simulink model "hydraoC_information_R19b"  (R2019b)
settings: Solver=VariableStepAuto  StartTime=0.0  StopTime=inf  FixedStep=1e-3  RelTol=1e-3
libraries: fl_lib x33, ee_lib x10, nesl_utility x6, simulink x2, sh_lib x1

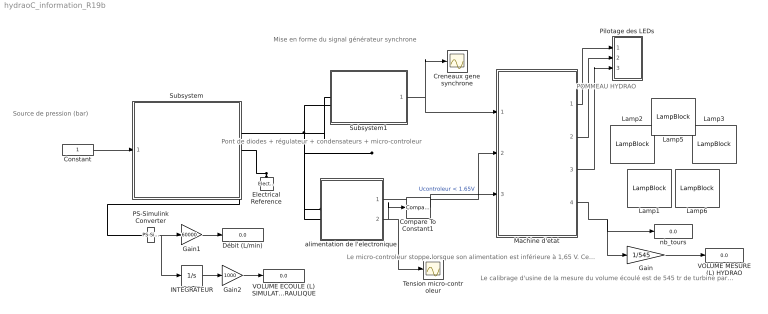
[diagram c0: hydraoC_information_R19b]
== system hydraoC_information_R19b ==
  note: POMMEAU HYDRAO
  note: Le calibrage d'usine de la mesure du volume écoulé est de 545 tr de turbine par litre.
  note: Mise en forme du signal générateur synchrone
  note: Pont de diodes + régulateur + condensateurs + micro-controleur
  note: Source de pression (bar)
  note: Le micro-controleur stoppe lorsque son alimentation est inférieure à 1,65 V. Cela entraine une perte des informations et un redémarrage en situation initiale au prochain écoulement
  Compare To Constant1 : simulink/Logic and Bit Operations/Compare To Constant  relop=<  const=1.65  OutDataTypeStr=boolean
  Constant : Constant
  Creneaux gene synchrone : Scope
  Débit (L/min) : Display
  Electrical Reference : fl_lib/Electrical/Electrical Elements/Electrical Reference
  Gain : Gain  Gain=1/545
  Gain1 : Gain  Gain=60000
  Gain2 : Gain  Gain=1000
  INTEGRATEUR : Integrator
  Lamp{1..3,5..6} (5 alike) : LampBlock
  Machine d'etat : Stateflow chart  TreatAsAtomicUnit=on
  PS-Simulink Converter : nesl_utility/PS-Simulink Converter  PhysicalDomain=network_engine_domain  SubClassName=ps_output  LeftPortType=input  RightPortType=output  PseudoPeriodic=off  Frequencies=[]  Unit=inherit  AffineConversion=off
  Pilotage des LEDs : Subsystem
  Subsystem : Subsystem
  Subsystem1 : Subsystem
  Tension micro-controleur : Scope
  VOLUME ECOULE (L) SIMULATION HYDRAULIQUE : Display
  VOLUME MESURE (L) HYDRAO : Display
  alimentation de l'electronique : Subsystem
  nb_tours : Display
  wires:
  Machine d'etat/2(LED_V) -> Pilotage des LEDs/2(V)
  Machine d'etat/3(LED_B) -> Pilotage des LEDs/3(B)
  Machine d'etat/1(LED_R) -> Pilotage des LEDs/1(R)
  Machine d'etat/4(nb_tours) -> nb_tours/1, Gain/1
  alimentation de l'electronique/2(Ucontroleur) -> Tension micro-controleur/1, Compare To Constant1/1
  Constant/1 -> Subsystem/1(In1)
  Subsystem1/1(Creneaux_gene_alt) -> Machine d'etat/1(creneau_gene), Creneaux gene synchrone/1
  alimentation de l'electronique/1(Image_Upuiss) -> Machine d'etat/2(image_Upuiss)
  Compare To Constant1/1 -> Machine d'etat/3(alim_LOW)  "Ucontroleur < 1.65V"
  Gain/1 -> VOLUME MESURE (L) HYDRAO/1
  PS-Simulink Converter/1 -> INTEGRATEUR/1, Gain1/1
  Gain1/1 -> Débit (L/min)/1
  Gain2/1 -> VOLUME ECOULE (L) SIMULATION HYDRAULIQUE/1
  INTEGRATEUR/1 -> Gain2/1
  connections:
  Subsystem/RConn1 -- alimentation de l'electronique/LConn1 -- Subsystem1/LConn1
  Electrical Reference/LConn1 -- Subsystem/RConn2 -- Subsystem1/LConn2 -- alimentation de l'electronique/LConn2
  Subsystem/RConn3 -- PS-Simulink Converter/LConn1

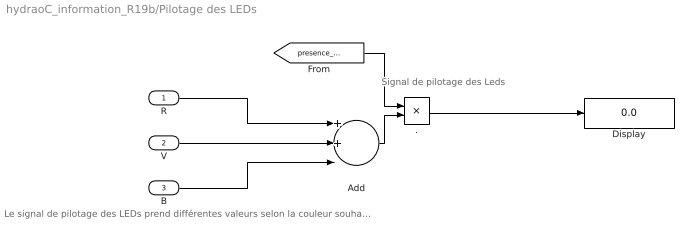
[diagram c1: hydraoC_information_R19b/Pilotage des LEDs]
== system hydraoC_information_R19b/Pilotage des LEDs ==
  note: Signal de pilotage des Leds
  note: Le signal de pilotage des LEDs prend différentes valeurs selon la couleur souhaitée Vmot est un booleen qui vaut 0L si la tension aux bornes du pont de diodes les LEDs ne peuvent s'éclairer que si le pont est alimenté donc si la turbine tourne
  R : Inport
  V : Inport  Port=2
  B : Inport  Port=3
  . : Product
  Add : Sum  Inputs=3
  Display : Display
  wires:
  B/1 -> Add/3
  ./1 -> Display/1
  R/1 -> Add/1
  V/1 -> Add/2
  Add/1 -> ./2
  [presence_Upuiss] -> ./1

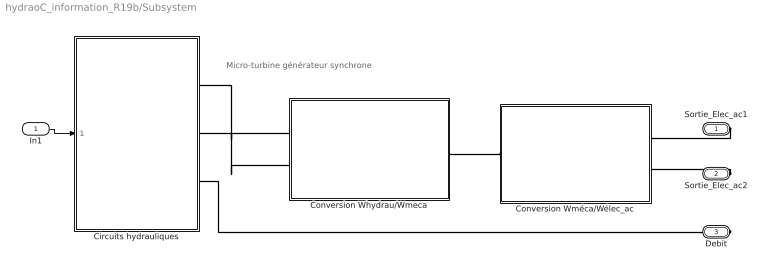
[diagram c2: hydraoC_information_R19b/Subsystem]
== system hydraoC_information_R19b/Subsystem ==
  note: Micro-turbine générateur synchrone
  In1 : Inport
  Circuits hydrauliques : Subsystem
  Conversion Whydrau/Wmeca : Subsystem
  Conversion Wméca/Wélec_ac : Subsystem
  Sortie_Elec_ac1 : PMIOPort  Side=Right
  Sortie_Elec_ac2 : PMIOPort  Port=2  Side=Right
  Debit : PMIOPort  Port=3  Side=Right
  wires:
  In1/1 -> Circuits hydrauliques/1(Pression source)
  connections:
  Sortie_Elec_ac1/RConn1 -- Conversion Wméca/Wélec_ac/RConn1
  Circuits hydrauliques/RConn2 -- Conversion Whydrau/Wmeca/LConn2
  Conversion Whydrau/Wmeca/RConn1 -- Conversion Wméca/Wélec_ac/LConn1
  Circuits hydrauliques/RConn1 -- Conversion Whydrau/Wmeca/LConn1
  Sortie_Elec_ac2/RConn1 -- Conversion Wméca/Wélec_ac/RConn2
  Circuits hydrauliques/RConn3 -- Debit/RConn1

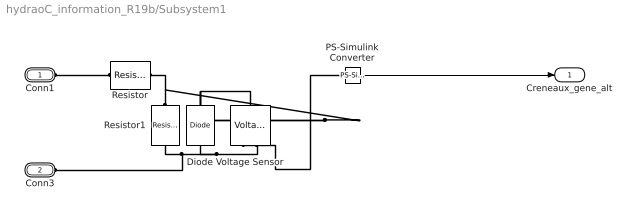
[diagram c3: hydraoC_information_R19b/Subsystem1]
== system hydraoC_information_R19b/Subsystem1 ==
  Diode : ee_lib/Semiconductors & Converters/Diode  ModelType=ee.enum.diode.modelType.pwl  Vf=0.6 V  Ron=0.3 Ohm  Goff=1e-8 S  prmExp=ee.enum.diode.expParam.useTwo  I12=[.0137, .545] A  V12=[.6, .7] V  IS=1e-12 A  ec=1  I1=0.0137 A  V1=0.6 V  RS=0 Ohm  Tmeas=25 degC  N_series=1  N_parallel=1  Rz=0.3 Ohm  BV=3 V  C_param=ee.enum.diode.capParam.fixed  CJ=5 pF  CJ0=5 pF  VJ=1 V  Mgrad=0.5  Vvec=[.1, 10, 100] V  Cvec=[3.5, 1, .4] pF  FC=0.5  Q_param=ee.enum.diode.recoveryParam.off  iRM=-7.15 A  iF=4 A  didt=-750 A/us  trr_factor=3  trr=115 ns  Qrr=1500 s*uA  TT=50 ns  tau=100 ns  T_param=ee.enum.diode.temperatureParam.off  IS_T2=1.25e-7 A  I1_T2=0.245 A  V1_T2=0.5 V  Tmeas2=125 degC  EG_param=ee.enum.diode.egapParam.material_si  EG=1.11 eV  XTI_param=ee.enum.diode.xtiParam.pn  XTI=3  dBVdT=0 V/K  Tdevice=25 degC  i_specify=off  i_priority=None  i=0 A  i_nominal_specify=off  i_nominal_unit=A  i_nominal_value=1  v_specify=off  v_priority=None  v=0 V  v_nominal_specify=off  v_nominal_unit=V  v_nominal_value=1  i_capacitor_specify=off  i_capacitor_priority=None  i_capacitor=0 A  i_capacitor_nominal_specify=off  i_capacitor_nominal_unit=A  i_capacitor_nominal_value=1  v_capacitor_specify=off  v_capacitor_priority=None  v_capacitor=0 V  v_capacitor_nominal_specify=off  v_capacitor_nominal_unit=V  v_capacitor_nominal_value=1  power_dissipated_specify=off  power_dissipated_priority=None  power_dissipated=0 W  power_dissipated_nominal_specify=off  power_dissipated_nominal_unit=W  power_dissipated_nominal_value=1  thermal_network_parameterization=ee.enum.thermalNetworkTopology.cauer  Rth=[0, 10] K/W  Rth_Foster=[4, 6] K/W  thermal_mass_parameterization=ee.enum.thermalNetwork.timeconstant  thermal_mass=[0, 1] J/K  thermal_mass_Foster=[1.5, 3] J/K  thermal_time_constant=[0, 10] s  thermal_time_constant_Foster=[6, 18] s  thermal_mass_initial_temperatures=[25, 25] degC
  PS-Simulink Converter : nesl_utility/PS-Simulink Converter  PhysicalDomain=network_engine_domain  SubClassName=ps_output  LeftPortType=input  RightPortType=output  PseudoPeriodic=off  Frequencies=[]  Unit=inherit  AffineConversion=off
  Resistor : fl_lib/Electrical/Electrical Elements/Resistor  R=10 kOhm  i_specify=off  i_priority=None  i=0 A  i_nominal_specify=off  i_nominal_unit=A  i_nominal_value=1  v_specify=off  v_priority=None  v=0 V  v_nominal_specify=off  v_nominal_unit=V  v_nominal_value=1
  Resistor1 : fl_lib/Electrical/Electrical Elements/Resistor  R=330 kOhm  i_specify=off  i_priority=None  i=0 A  i_nominal_specify=off  i_nominal_unit=A  i_nominal_value=1  v_specify=off  v_priority=None  v=0 V  v_nominal_specify=off  v_nominal_unit=V  v_nominal_value=1
  Voltage Sensor : fl_lib/Electrical/Electrical Sensors/Voltage Sensor
  Conn1 : PMIOPort  Side=Left
  Conn3 : PMIOPort  Port=2  Side=Left
  Creneaux_gene_alt : Outport
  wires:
  PS-Simulink Converter/1 -> Creneaux_gene_alt/1
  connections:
  Resistor1/LConn1 -- Resistor/RConn1 -- Voltage Sensor/LConn1 -- Diode/RConn1
  Voltage Sensor/RConn2 -- Diode/LConn1 -- Conn3/RConn1 -- Resistor1/RConn1
  Resistor/LConn1 -- Conn1/RConn1
  PS-Simulink Converter/LConn1 -- Voltage Sensor/RConn1

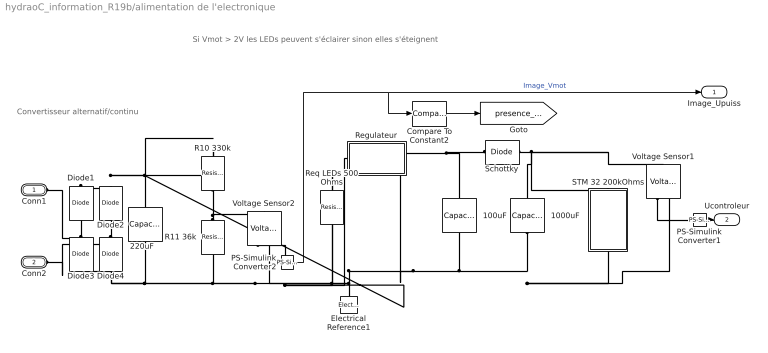
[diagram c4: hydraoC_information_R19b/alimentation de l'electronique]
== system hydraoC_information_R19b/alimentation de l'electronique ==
  note: Convertisseur alternatif/continu
  note: Si Vmot > 2V les LEDs peuvent s'éclairer sinon elles s'éteignent
  " 1000uF" : ee_lib/Passive/Capacitor  cap_option=0  c=1000 uF  Cvec=[1e-05, 1e-06] F  Vvec=[0, 10] V  CV_table_symmetry=1  f_vec=[1, 10] kHz  DFext_vec=[.8, 1.2]  C_tol=5  enable_C_tol=0  tol_distribution=1  nSigma=4  r=1e-6 Ohm  g=0 1/Ohm  averaging_period=0 s  enable_operating_limits=0  operating_limit_action=2  max_working_voltage_range=[-25, 25] V  power_rating=1 W  enable_faults=0  fault_action=1  Cscale_faulted=100  R_faulted=1e-3 Ohm  G_faulted=0 1/Ohm  tau_fault=1e-3 s  enable_temporal_fault=0  t_fault=1 s  enable_behavioral_fault=0  max_permissible_voltage_range=[-100, 100] V  t_fail_on_voltage=1 s  i_specify=off  i_priority=None  i=0 A  i_nominal_specify=off  i_nominal_unit=A  i_nominal_value=1  v_specify=off  v_priority=None  v=0 V  v_nominal_specify=off  v_nominal_unit=V  v_nominal_value=1  vc_specify=off  vc_priority=High  vc=0 V  vc_nominal_specify=off  vc_nominal_unit=V  vc_nominal_value=1
  " 100uF" : ee_lib/Passive/Capacitor  cap_option=0  c=100 uF  Cvec=[1e-05, 1e-06] F  Vvec=[0, 10] V  CV_table_symmetry=1  f_vec=[1, 10] kHz  DFext_vec=[.8, 1.2]  C_tol=5  enable_C_tol=0  tol_distribution=1  nSigma=4  r=1e-6 Ohm  g=0 1/Ohm  averaging_period=0 s  enable_operating_limits=0  operating_limit_action=2  max_working_voltage_range=[-25, 25] V  power_rating=1 W  enable_faults=0  fault_action=1  Cscale_faulted=100  R_faulted=1e-3 Ohm  G_faulted=0 1/Ohm  tau_fault=1e-3 s  enable_temporal_fault=0  t_fault=1 s  enable_behavioral_fault=0  max_permissible_voltage_range=[-100, 100] V  t_fail_on_voltage=1 s  i_specify=off  i_priority=None  i=0 A  i_nominal_specify=off  i_nominal_unit=A  i_nominal_value=1  v_specify=off  v_priority=None  v=0 V  v_nominal_specify=off  v_nominal_unit=V  v_nominal_value=1  vc_specify=off  vc_priority=High  vc=0 V  vc_nominal_specify=off  vc_nominal_unit=V  vc_nominal_value=1
  " 220uF" : ee_lib/Passive/Capacitor  cap_option=0  c=220 uF  Cvec=[1e-05, 1e-06] F  Vvec=[0, 10] V  CV_table_symmetry=1  f_vec=[1, 10] kHz  DFext_vec=[.8, 1.2]  C_tol=5  enable_C_tol=0  tol_distribution=1  nSigma=4  r=1e-6 Ohm  g=0 1/Ohm  averaging_period=0 s  enable_operating_limits=0  operating_limit_action=2  max_working_voltage_range=[-25, 25] V  power_rating=1 W  enable_faults=0  fault_action=1  Cscale_faulted=100  R_faulted=1e-3 Ohm  G_faulted=0 1/Ohm  tau_fault=1e-3 s  enable_temporal_fault=0  t_fault=1 s  enable_behavioral_fault=0  max_permissible_voltage_range=[-100, 100] V  t_fail_on_voltage=1 s  i_specify=off  i_priority=None  i=0 A  i_nominal_specify=off  i_nominal_unit=A  i_nominal_value=1  v_specify=off  v_priority=None  v=0 V  v_nominal_specify=off  v_nominal_unit=V  v_nominal_value=1  vc_specify=off  vc_priority=High  vc=0 V  vc_nominal_specify=off  vc_nominal_unit=V  vc_nominal_value=1
  Compare To Constant2 : simulink/Logic and Bit Operations/Compare To Constant  relop=>  const=0.2  OutDataTypeStr=boolean
  Diode{1..4} (4 alike) : fl_lib/Electrical/Electrical Elements/Diode  Vf=0.3 V  Ron=1 Ohm  Goff=1e-8 1/Ohm  i_specify=off  i_priority=None  i=0 A  i_nominal_specify=off  i_nominal_unit=A  i_nominal_value=1  v_specify=off  v_priority=None  v=0 V  v_nominal_specify=off  v_nominal_unit=V  v_nominal_value=1
  Electrical Reference1 : fl_lib/Electrical/Electrical Elements/Electrical Reference
  PS-Simulink Converter1 : nesl_utility/PS-Simulink Converter  PhysicalDomain=network_engine_domain  SubClassName=ps_output  LeftPortType=input  RightPortType=output  PseudoPeriodic=off  Frequencies=[]  Unit=inherit  AffineConversion=off
  PS-Simulink Converter2 : nesl_utility/PS-Simulink Converter  PhysicalDomain=network_engine_domain  SubClassName=ps_output  LeftPortType=input  RightPortType=output  PseudoPeriodic=off  Frequencies=[]  Unit=inherit  AffineConversion=off
  R10 330k : fl_lib/Electrical/Electrical Elements/Resistor  R=330 kOhm  i_specify=off  i_priority=None  i=0 A  i_nominal_specify=off  i_nominal_unit=A  i_nominal_value=1  v_specify=off  v_priority=None  v=0 V  v_nominal_specify=off  v_nominal_unit=V  v_nominal_value=1
  R11 36k : fl_lib/Electrical/Electrical Elements/Resistor  R=36 kOhm  i_specify=off  i_priority=None  i=0 A  i_nominal_specify=off  i_nominal_unit=A  i_nominal_value=1  v_specify=off  v_priority=None  v=0 V  v_nominal_specify=off  v_nominal_unit=V  v_nominal_value=1
  Regulateur : Subsystem
  Req LEDs 500 Ohms : fl_lib/Electrical/Electrical Elements/Resistor  R=500 Ohm  i_specify=off  i_priority=None  i=0 A  i_nominal_specify=off  i_nominal_unit=A  i_nominal_value=1  v_specify=off  v_priority=None  v=0 V  v_nominal_specify=off  v_nominal_unit=V  v_nominal_value=1
  STM 32 200kOhms : Subsystem
  Schottky : ee_lib/Semiconductors & Converters/Diode  ModelType=ee.enum.diode.modelType.pwl  Vf=0.3 V  Ron=0.3 Ohm  Goff=1e-8 S  prmExp=ee.enum.diode.expParam.useTwo  I12=[.0137, .545] A  V12=[.6, .7] V  IS=1e-12 A  ec=1  I1=0.0137 A  V1=0.6 V  RS=0 Ohm  Tmeas=25 degC  N_series=1  N_parallel=1  Rz=0.3 Ohm  BV=100 V  C_param=ee.enum.diode.capParam.fixed  CJ=5 pF  CJ0=5 pF  VJ=1 V  Mgrad=0.5  Vvec=[.1, 10, 100] V  Cvec=[3.5, 1, .4] pF  FC=0.5  Q_param=ee.enum.diode.recoveryParam.off  iRM=-7.15 A  iF=4 A  didt=-750 A/us  trr_factor=3  trr=115 ns  Qrr=1500 s*uA  TT=50 ns  tau=100 ns  T_param=ee.enum.diode.temperatureParam.off  IS_T2=1.25e-7 A  I1_T2=0.245 A  V1_T2=0.5 V  Tmeas2=125 degC  EG_param=ee.enum.diode.egapParam.material_si  EG=1.11 eV  XTI_param=ee.enum.diode.xtiParam.pn  XTI=3  dBVdT=0 V/K  Tdevice=25 degC  i_specify=off  i_priority=None  i=0 A  i_nominal_specify=off  i_nominal_unit=A  i_nominal_value=1  v_specify=off  v_priority=None  v=0 V  v_nominal_specify=off  v_nominal_unit=V  v_nominal_value=1  i_capacitor_specify=off  i_capacitor_priority=None  i_capacitor=0 A  i_capacitor_nominal_specify=off  i_capacitor_nominal_unit=A  i_capacitor_nominal_value=1  v_capacitor_specify=off  v_capacitor_priority=None  v_capacitor=0 V  v_capacitor_nominal_specify=off  v_capacitor_nominal_unit=V  v_capacitor_nominal_value=1  power_dissipated_specify=off  power_dissipated_priority=None  power_dissipated=0 W  power_dissipated_nominal_specify=off  power_dissipated_nominal_unit=W  power_dissipated_nominal_value=1  thermal_network_parameterization=ee.enum.thermalNetworkTopology.cauer  Rth=[0, 10] K/W  Rth_Foster=[4, 6] K/W  thermal_mass_parameterization=ee.enum.thermalNetwork.timeconstant  thermal_mass=[0, 1] J/K  thermal_mass_Foster=[1.5, 3] J/K  thermal_time_constant=[0, 10] s  thermal_time_constant_Foster=[6, 18] s  thermal_mass_initial_temperatures=[25, 25] degC
  Voltage Sensor1 : fl_lib/Electrical/Electrical Sensors/Voltage Sensor
  Voltage Sensor2 : fl_lib/Electrical/Electrical Sensors/Voltage Sensor
  Conn1 : PMIOPort  Side=Left
  Conn2 : PMIOPort  Port=2  Side=Left
  Image_Upuiss : Outport
  Ucontroleur : Outport  Port=2
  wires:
  PS-Simulink Converter1/1 -> Ucontroleur/1
  PS-Simulink Converter2/1 -> Compare To Constant2/1, Image_Upuiss/1  "Image_Vmot"
  Compare To Constant2/1 -> [presence_Upuiss]
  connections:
  " 1000uF"/RConn1 -- " 220uF"/RConn1 -- Diode4/LConn1 -- Diode3/LConn1 -- R11 36k/RConn1 -- Voltage Sensor2/RConn2 -- Req LEDs 500 Ohms/RConn1 -- Electrical Reference1/LConn1 -- Regulateur/RConn2 -- " 100uF"/RConn1 -- Voltage Sensor1/RConn2 -- STM 32 200kOhms/RConn1
  Schottky/RConn1 -- " 1000uF"/LConn1 -- STM 32 200kOhms/LConn1 -- Voltage Sensor1/LConn1
  Diode4/RConn1 -- Diode2/LConn1 -- Conn2/RConn1
  Diode1/RConn1 -- R10 330k/LConn1 -- Req LEDs 500 Ohms/LConn1 -- Regulateur/LConn1 -- " 220uF"/LConn1 -- Diode2/RConn1
  Voltage Sensor1/RConn1 -- PS-Simulink Converter1/LConn1
  Regulateur/RConn1 -- " 100uF"/LConn1 -- Schottky/LConn1
  Diode3/RConn1 -- Diode1/LConn1 -- Conn1/RConn1
  PS-Simulink Converter2/LConn1 -- Voltage Sensor2/RConn1
  R11 36k/LConn1 -- Voltage Sensor2/LConn1 -- R10 330k/RConn1

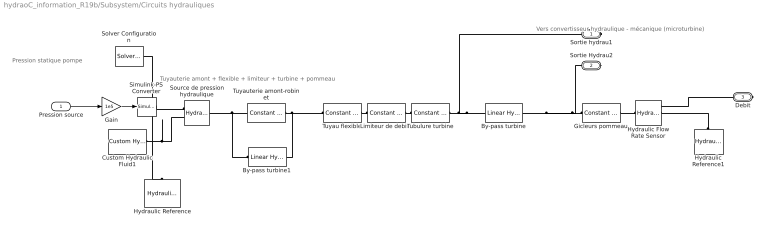
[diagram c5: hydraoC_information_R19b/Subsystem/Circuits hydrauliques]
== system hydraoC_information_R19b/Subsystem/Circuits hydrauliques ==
  note: Pression statique pompe
  note: Tuyauterie amont + flexible + limiteur + turbine + pommeau
  note: Vers convertisseur hydraulique - mécanique (microturbine)
  Pression source : Inport
  By-pass turbine : fl_lib/Hydraulic/Hydraulic Elements/Linear Hydraulic Resistance  Commented=on  resistance=1e0 Pa/(m^3/s)  q_specify=off  q_priority=None  q=0.001 m^3/s  q_nominal_specify=off  q_nominal_unit=m^3/s  q_nominal_value=1  p_specify=off  p_priority=None  p=0 Pa  p_nominal_specify=off  p_nominal_unit=Pa  p_nominal_value=1
  By-pass turbine1 : fl_lib/Hydraulic/Hydraulic Elements/Linear Hydraulic Resistance  Commented=on  resistance=1e0 Pa/(m^3/s)  q_specify=off  q_priority=None  q=0.001 m^3/s  q_nominal_specify=off  q_nominal_unit=m^3/s  q_nominal_value=1  p_specify=off  p_priority=None  p=0 Pa  p_nominal_specify=off  p_nominal_unit=Pa  p_nominal_value=1
  Custom Hydraulic Fluid1 : fl_lib/Hydraulic/Hydraulic Utilities/Custom Hydraulic Fluid  density=994 kg/m^3  viscosity_kin=7.35e-7 m^2/s  bulk=8e8 Pa  alpha=0.005  range_error=2
  Gain : Gain  Gain=1e5
  Gicleurs pommeau : fl_lib/Hydraulic/Hydraulic Elements/Constant Area Hydraulic Orifice  area=20e-6 m^2  C_d=0.4  lam_spec=2  B_lam=0.999  Re_cr=1e0  q_specify=off  q_priority=None  q=0.001 m^3/s  q_nominal_specify=off  q_nominal_unit=m^3/s  q_nominal_value=1  p_specify=off  p_priority=None  p=0 Pa  p_nominal_specify=off  p_nominal_unit=Pa  p_nominal_value=1
  Hydraulic Flow Rate Sensor : fl_lib/Hydraulic/Hydraulic Sensors/Hydraulic Flow Rate Sensor
  Hydraulic Reference : fl_lib/Hydraulic/Hydraulic Elements/Hydraulic Reference
  Hydraulic Reference1 : fl_lib/Hydraulic/Hydraulic Elements/Hydraulic Reference
  Limiteur de debit4 : fl_lib/Hydraulic/Hydraulic Elements/Constant Area Hydraulic Orifice  area=20e-6 m^2  C_d=.5  lam_spec=2  B_lam=0.999  Re_cr=1e0  q_specify=off  q_priority=None  q=0.001 m^3/s  q_nominal_specify=off  q_nominal_unit=m^3/s  q_nominal_value=1  p_specify=off  p_priority=None  p=0 Pa  p_nominal_specify=off  p_nominal_unit=Pa  p_nominal_value=1
  Simulink-PS Converter : nesl_utility/Simulink-PS Converter  PhysicalDomain=network_engine_domain  SubClassName=ps_input  LeftPortType=input  RightPortType=output  PseudoPeriodic=off  Frequencies=[]  NoiseDistribution=none  NoiseParameters=[]  Unit=1  AffineConversion=off  FilteringAndDerivatives=provide  SimscapeFilterOrder=1  InputFilterTimeConstant=0.001  UdotUserProvided=0
  Solver Configuration : nesl_utility/Solver Configuration  PhysicalDomain=network_engine_domain  SubClassName=solver  LeftPortType=input  RightPortType=generic  Tones=[]  Harmonics=[]  SimulateNoise=off  Profile=off  UseLocalSampling=off  EnableSwitchedLinearOptims=on  FrequencyDomain=off  UseCCode=off  RelTol=0.001  AbsTol=1e-06  MinStep=1e-09  ToWorkspace=off  RevertToSquareIcSolve=off  NumHomotopyIterations=100  PhasorMode=off  PhasorModeNumHarmonics=1  DoDC=off  ResidualTolerance=1e-9  UseLocalSolver=off  LocalSolverChoice=NE_BACKWARD_EULER_ADVANCER  LocalSolverSampleTime=0.001  DoFixedCost=off  MaxNonlinIter=3  MaxModeIter=2  LinearAlgebra=Sparse  EquationFormulation=NE_TIME_EF  DelaysMemoryBudget=1024  AutomaticFiltering=on  FilteringTimeConstant=0.001  PartitionStorageMethod=AS_NEEDED  PartitionMemoryBudget=1024  PartitionMethod=FAST
  Source de pression hydraulique : fl_lib/Hydraulic/Hydraulic Sources/Hydraulic Pressure Source
  Tubulure turbine : fl_lib/Hydraulic/Hydraulic Elements/Constant Area Hydraulic Orifice  area=12.7e-6 m^2  C_d=0.81  lam_spec=2  B_lam=0.999  Re_cr=1e0  q_specify=off  q_priority=None  q=0.001 m^3/s  q_nominal_specify=off  q_nominal_unit=m^3/s  q_nominal_value=1  p_specify=off  p_priority=None  p=0 Pa  p_nominal_specify=off  p_nominal_unit=Pa  p_nominal_value=1
  Tuyau flexible : fl_lib/Hydraulic/Hydraulic Elements/Constant Area Hydraulic Orifice  area=41e-6 m^2  C_d=0.25  lam_spec=2  B_lam=2000  Re_cr=1e0  q_specify=off  q_priority=None  q=0.001 m^3/s  q_nominal_specify=off  q_nominal_unit=m^3/s  q_nominal_value=1  p_specify=off  p_priority=None  p=0 Pa  p_nominal_specify=off  p_nominal_unit=Pa  p_nominal_value=1
  Tuyauterie amont-robinet : fl_lib/Hydraulic/Hydraulic Elements/Constant Area Hydraulic Orifice  area=113e-6 m^2  C_d=0.134  lam_spec=2  B_lam=0.999  Re_cr=1e0  q_specify=off  q_priority=None  q=0.001 m^3/s  q_nominal_specify=off  q_nominal_unit=m^3/s  q_nominal_value=1  p_specify=off  p_priority=None  p=0 Pa  p_nominal_specify=off  p_nominal_unit=Pa  p_nominal_value=1
  Sortie hydrau1 : PMIOPort  Side=Right
  Sortie Hydrau2 : PMIOPort  Port=2  Side=Right
  Debit : PMIOPort  Port=3  Side=Right
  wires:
  Gain/1 -> Simulink-PS Converter/1
  Pression source/1 -> Gain/1
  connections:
  Custom Hydraulic Fluid1/RConn1 -- Solver Configuration/RConn1 -- Source de pression hydraulique/RConn2 -- Hydraulic Reference/LConn1
  Simulink-PS Converter/RConn1 -- Source de pression hydraulique/RConn1
  By-pass turbine1/LConn1 -- Tuyauterie amont-robinet/LConn1 -- Source de pression hydraulique/LConn1
  Gicleurs pommeau/RConn1 -- Hydraulic Flow Rate Sensor/LConn1
  Gicleurs pommeau/LConn1 -- By-pass turbine/RConn1 -- Sortie Hydrau2/RConn1
  Tuyauterie amont-robinet/RConn1 -- By-pass turbine1/RConn1 -- Tuyau flexible/LConn1
  Tubulure turbine/RConn1 -- By-pass turbine/LConn1 -- Sortie hydrau1/RConn1
  Hydraulic Reference1/LConn1 -- Hydraulic Flow Rate Sensor/RConn2
  Hydraulic Flow Rate Sensor/RConn1 -- Debit/RConn1
  Tuyau flexible/RConn1 -- Limiteur de debit4/LConn1
  Tubulure turbine/LConn1 -- Limiteur de debit4/RConn1

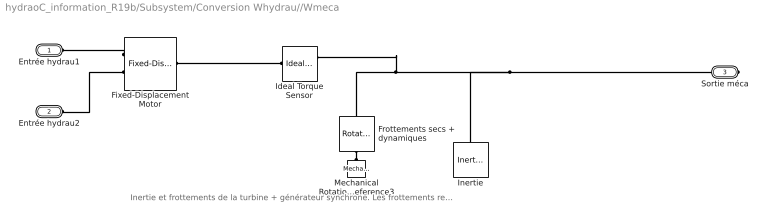
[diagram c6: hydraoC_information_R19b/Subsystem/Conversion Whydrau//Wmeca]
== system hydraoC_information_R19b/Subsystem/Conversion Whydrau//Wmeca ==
  note: Inertie et frottements de la turbine + générateur synchrone. Les frottements représentent les pertes mécaniques
  Fixed-Displacement Motor : sh_lib/Pumps and Motors/Fixed-Displacement Motor  D=0.3 cm^3/rad  loss_spec=1  w_nominal=300 rad/s  pr_nominal=100e5 Pa  visc_nominal=1e-6 m^2/s  dens_nominal=997 kg/m^3  efficiency_vol=0.92  no_load_torque=1e-4 N*m  torque_pressure_coeff=1e-7 N*m/Pa  p_diff_eff_TLU=[100000, 1000000, 2000000] Pa  omega_eff_TLU=[25, 50, 100, 200, 300, 400] rad/s  vol_eff_TLU=[.816, .908, .954, .977, .981, .984; .325, .663, .831, .916, .925, .946; .137, .568, .78, .892, .893, .91]  mech_eff_TLU=[.996, .996, .996, .996, .996, .996; .988, .989, .989, .989, .989, .99; .981, .981, .982, .982, .983, .984]  p_diff_loss_TLU=[100000, 1000000, 2000000] Pa  omega_loss_TLU=[25, 50, 100, 200, 300, 400] rad/s  vol_loss_TLU=[.0282, .0253, .0241, .0235, .0291, .0325; .2596, .1271, .1017, .0917, .1216, .1142; .7874, .1901, .141, .1211, .1797, .1978] * 1e-3 m^3/s  mech_loss_TLU=[.002, .002, .002, .002, .002, .002; .06, .055, .055, .055, .055, .05; .19, .19, .18, .18, .17, .16] N*m  pressure_threshold=1e5 Pa  omega_threshold=10 rad/s  quadrant_check=0  pressure_check=0  min_valid_pressure=0 Pa  vol_eff_min=1e-3  vol_eff_max=1  mech_eff_min=1e-3  mech_eff_max=1
  Frottements secs + dynamiques : fl_lib/Mechanical/Rotational Elements/Rotational Friction  brkwy_trq=1.5e-4 N*m  brkwy_vel=0.1 rad/s  Col_trq=1.5e-4 N*m  visc_coef=2.7e-7 N*m/(rad/s)  w_specify=off  w_priority=None  w=0 rad/s  w_nominal_specify=off  w_nominal_unit=rad/s  w_nominal_value=1  t_specify=off  t_priority=None  t=0 N*m  t_nominal_specify=off  t_nominal_unit=N*m  t_nominal_value=1
  Ideal Torque Sensor : fl_lib/Mechanical/Mechanical Sensors/Ideal Torque Sensor
  Inertie : fl_lib/Mechanical/Rotational Elements/Inertia  inertia=1.3e-8 kg*m^2  w_specify=off  w_priority=High  w=0 rad/s  w_nominal_specify=off  w_nominal_unit=rad/s  w_nominal_value=1  t_specify=off  t_priority=None  t=0 N*m  t_nominal_specify=off  t_nominal_unit=N*m  t_nominal_value=1
  Mechanical Rotational Reference3 : fl_lib/Mechanical/Rotational Elements/Mechanical Rotational Reference
  Entrée hydrau1 : PMIOPort  Side=Left
  Entrée hydrau2 : PMIOPort  Port=2  Side=Left
  Sortie méca : PMIOPort  Port=3  Side=Right
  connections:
  Fixed-Displacement Motor/LConn1 -- Entrée hydrau1/RConn1
  Sortie méca/RConn1 -- Frottements secs + dynamiques/LConn1 -- Ideal Torque Sensor/RConn1 -- Inertie/LConn1
  Ideal Torque Sensor/LConn1 -- Fixed-Displacement Motor/RConn1
  Frottements secs + dynamiques/RConn1 -- Mechanical Rotational Reference3/LConn1
  Entrée hydrau2/RConn1 -- Fixed-Displacement Motor/LConn2

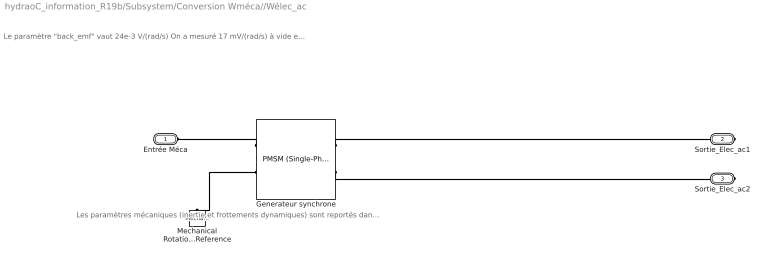
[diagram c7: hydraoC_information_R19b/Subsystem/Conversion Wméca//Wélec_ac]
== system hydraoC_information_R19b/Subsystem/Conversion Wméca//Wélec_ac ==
  note: Les paramètres mécaniques (inertie et frottements dynamiques) sont reportés dans le sous-système Conversion Whydrau/Wmeca
  note: Le paramètre "back_emf" vaut 24e-3 V/(rad/s) On a mesuré 17 mV/(rad/s) à vide et on multiplie par racine de 2 car "Back EMF est donnée en valeur max
  Generateur synchrone : ee_lib/Electromechanical/Permanent Magnet/PMSM (Single-Phase)  nPolePairs=1  pmflux_param=2  pm_flux_linkage=0.2 Wb  back_emf_constant=24e-3 V/(rad/s)  L=10 mH  Rs=146 Ohm  J=1e-12 kg*m^2  lam=1e-12 N*m/(rad/s)  pos_standstill=0 deg  i_specify=off  i_priority=High  i=0 A  i_nominal_specify=off  i_nominal_unit=A  i_nominal_value=1  torque_specify=off  torque_priority=None  torque=0 N*m  torque_nominal_specify=off  torque_nominal_unit=N*m  torque_nominal_value=1  angular_velocity_specify=off  angular_velocity_priority=High  angular_velocity=0 rpm  angular_velocity_nominal_specify=off  angular_velocity_nominal_unit=rpm  angular_velocity_nominal_value=1  angular_position_specify=off  angular_position_priority=High  angular_position=0 deg  angular_position_nominal_specify=off  angular_position_nominal_unit=deg  angular_position_nominal_value=1
  Mechanical Rotational Reference : fl_lib/Mechanical/Rotational Elements/Mechanical Rotational Reference
  Entrée Méca : PMIOPort  Side=Left
  Sortie_Elec_ac1 : PMIOPort  Port=2  Side=Right
  Sortie_Elec_ac2 : PMIOPort  Port=3  Side=Right
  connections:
  Generateur synchrone/RConn2 -- Mechanical Rotational Reference/LConn1
  Generateur synchrone/RConn1 -- Entrée Méca/RConn1
  Generateur synchrone/LConn2 -- Sortie_Elec_ac2/RConn1
  Generateur synchrone/LConn1 -- Sortie_Elec_ac1/RConn1

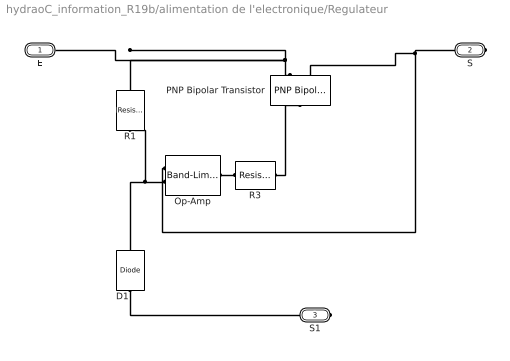
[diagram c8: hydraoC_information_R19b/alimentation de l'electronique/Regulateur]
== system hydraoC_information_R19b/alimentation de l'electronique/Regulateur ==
  D1 : ee_lib/Semiconductors & Converters/Diode  ModelType=ee.enum.diode.modelType.pwl  Vf=0.6 V  Ron=10 Ohm  Goff=1e-08 S  prmExp=ee.enum.diode.expParam.useTwo  I12="[  0.07 1.5 ] A"  V12="[  0.7 0.8 ] V"  IS=1e-14 A  ec=1  I1=0.0137 A  V1=0.6 V  RS=0.01 Ohm  Tmeas=25 degC  N_series=1  N_parallel=1  Rz=1 Ohm  BV=3.3 V  C_param=ee.enum.diode.capParam.fixed  CJ=5 pF  CJ0=5 pF  VJ=1 V  Mgrad=0.5  Vvec="[  0.1 10 100 ] V"  Cvec="[  3.5 1 0.4 ] pF"  FC=0.5  Q_param=ee.enum.diode.recoveryParam.off  iRM=-7.15 A  iF=4 A  didt=-750 A/us  trr_factor=3  trr=115 ns  Qrr=1500 s*uA  TT=50 ns  tau=100 ns  T_param=ee.enum.diode.temperatureParam.off  IS_T2=1.25e-7 A  I1_T2=0.245 A  V1_T2=0.5 V  Tmeas2=125 degC  EG_param=ee.enum.diode.egapParam.material_si  EG=1.11 eV  XTI_param=ee.enum.diode.xtiParam.pn  XTI=3  dBVdT=0 V/K  Tdevice=25 degC  i_specify=off  i_priority=None  i=0 A  i_nominal_specify=off  i_nominal_unit=A  i_nominal_value=1  v_specify=off  v_priority=None  v=0 V  v_nominal_specify=off  v_nominal_unit=V  v_nominal_value=1  i_capacitor_specify=off  i_capacitor_priority=High  i_capacitor=0 A  i_capacitor_nominal_specify=off  i_capacitor_nominal_unit=A  i_capacitor_nominal_value=1  v_capacitor_specify=off  v_capacitor_priority=None  v_capacitor=0 V  v_capacitor_nominal_specify=off  v_capacitor_nominal_unit=V  v_capacitor_nominal_value=1  power_dissipated_specify=off  power_dissipated_priority=None  power_dissipated=0 W  power_dissipated_nominal_specify=off  power_dissipated_nominal_unit=W  power_dissipated_nominal_value=1  thermal_network_parameterization=ee.enum.thermalNetworkTopology.cauer  Rth=[0, 10] K/W  Rth_Foster=[4, 6] K/W  thermal_mass_parameterization=ee.enum.thermalNetwork.timeconstant  thermal_mass=[0, 1] J/K  thermal_mass_Foster=[1.5, 3] J/K  thermal_time_constant=[0, 10] s  thermal_time_constant_Foster=[6, 18] s  thermal_mass_initial_temperatures=[25, 25] degC
  Op-Amp : ee_lib/Integrated Circuits/Band-Limited Op-Amp  A=100000  Rin=2 MOhm  Rout=100 Ohm  Vmin=-0.5 V  Vmax=30 V  Vdotmax=1e6 V/s  f=2 MHz  V0=0 V
  PNP Bipolar Transistor : ee_lib/Semiconductors & Converters/PNP Bipolar Transistor  parameterization=1  prmDatasheet=1  prmEquCoeff=1  BF=100  IS=1e-14 A  VAF=200 V  hfe=100  hoe=50e-6 1/Ohm  Ic_h=-1 A  Vce_h=-15 V  V1=-0.55 V  I1=-1 mA  BR=0.1  Tmeas=25 degC  RC=0.01 Ohm  RE=1e-4 Ohm  RB=1 Ohm  C_BC=5 pF  C_BE=5 pF  TF=0 us  TR=0 us  hfe_T2=125  XTB=0  V1_T2=-0.45 V  I1_T2=-0.5 mA  Tmeas2=125 degC  EG=1.11 eV  XTI=3  ec=1  TdeviceDatasheet=25 degC  TdeviceEquCoeff=25 degC  thermal_network_parameterization=ee.enum.thermalNetworkTopology.cauer  Rth=[0, 10] K/W  Rth_Foster=[4, 6] K/W  thermal_mass_parameterization=ee.enum.thermalNetwork.timeconstant  thermal_mass=[0, 1] J/K  thermal_mass_Foster=[1.5, 3] J/K  thermal_time_constant=[0, 10] s  thermal_time_constant_Foster=[6, 18] s  thermal_mass_initial_temperatures=[25, 25] degC
  R1 : fl_lib/Electrical/Electrical Elements/Resistor  R=1 kOhm  i_specify=off  i_priority=High  i=0 A  i_nominal_specify=off  i_nominal_unit=A  i_nominal_value=1  v_specify=off  v_priority=High  v=0 V  v_nominal_specify=off  v_nominal_unit=V  v_nominal_value=1
  R3 : fl_lib/Electrical/Electrical Elements/Resistor  R=10 kOhm  i_specify=off  i_priority=High  i=0 A  i_nominal_specify=off  i_nominal_unit=A  i_nominal_value=1  v_specify=off  v_priority=High  v=0 V  v_nominal_specify=off  v_nominal_unit=V  v_nominal_value=1
  E : PMIOPort  Side=Left
  S : PMIOPort  Port=2  Side=Right
  S1 : PMIOPort  Port=3  Side=Right
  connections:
  R3/RConn1 -- PNP Bipolar Transistor/LConn1
  Op-Amp/LConn2 -- D1/RConn1 -- R1/RConn1
  Op-Amp/RConn1 -- R3/LConn1
  PNP Bipolar Transistor/RConn1 -- R1/LConn1 -- E/RConn1
  Op-Amp/LConn1 -- PNP Bipolar Transistor/RConn2 -- S/RConn1
  D1/LConn1 -- S1/RConn1

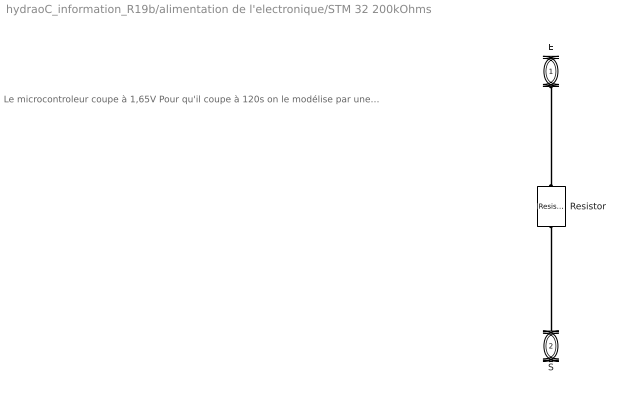
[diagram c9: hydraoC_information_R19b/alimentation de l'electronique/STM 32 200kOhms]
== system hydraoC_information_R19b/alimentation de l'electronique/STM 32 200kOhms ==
  note: Le microcontroleur coupe à 1,65V Pour qu'il coupe à 120s on le modélise par une résistance de 200k ce qui donne un courant d'alim de 3/200k = 15 microA Sachant que la conso du microC est de 88microA par MHz en RUN on en déduit qu'il est cadencé à 15/88 = 0,170 MHz ?
  Resistor : ee_lib/Passive/Resistor  R=200 kOhm  R_tol=5  enable_R_tol=0  tol_distribution=1  nSigma=4  enable_operating_limits=0  operating_limit_action=2  max_working_voltage=100 V  power_rating=1 W  enable_faults=0  fault_action=1  R_faulted=inf Ohm  enable_temporal_fault=0  t_fault=1 s  enable_behavioral_fault=0  max_permissible_current=1 A  t_fail_on_current=1 s  noise_mode=0  sample_time=1e-3 s  repeatability=1  auto_seed=3499211588  user_seed=0  Tdevice=25 degC  alpha=3.93e-3 1/K  Tmeas=25 degC  thermal_mass=100 J/K  power_derating_T1=70 degC  power_derating_T2=155 degC  operating_temperature_range_vec=[-50, 150] degC  temperature_specify=off  temperature_priority=High  temperature=298.15 K  temperature_nominal_specify=off  temperature_nominal_unit=K  temperature_nominal_value=1
  E : PMIOPort  Side=Left
  S : PMIOPort  Port=2  Side=Right
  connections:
  S/RConn1 -- Resistor/RConn1
  E/RConn1 -- Resistor/LConn1

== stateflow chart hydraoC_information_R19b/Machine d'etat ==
  state Pommeau
    during :
    LED_R=bitand(RGB, 0b100);
    LED_V=bitand(RGB, 0b010);
    LED_B=bitand(RGB, 0b001);
    state <!DOCTYPE HTML PUBLIC "-//W3C//DTD HTML 4.0//EN" "http://www.w3.org/TR/REC-html40/strict.dtd"> [group]
      <html><head><meta name="qrichtext" content="1" /><style type="text/css">
      p, li { white-space: pre-wrap; }
      </style></head><body align="left" style=" font-family:'Helvetica'; font-size:12px; font-weight:400; font-style:normal;">
      <p align="left" style=" margin-top:0px; margin-bottom:0px; margin-left:0px; margin-right:0px; -qt-block-indent:0; text-indent:0px;"><span style=" font-size:12px; background-color:#00ff00;">Machine d'état avec états composites</span></p></body></html>
    state Gestion_signaux_et_evenements [parallel]
      state Gestion_signaux_et_evenements_
        entry :
        nb_tours=0; nb_tours_prec=0;
        image_Upuiss_prec=0;
        alim_LOW_prec=false; signal_gene_prec=false;
        vol_eau_sup_10l=false; vol_eau_sup_20l=false;
        vol_eau_sup_30l=false; vol_eau_sup_40l=false;
        during :
        %Traitement créneaux génératrice
        if creneau_gene > 1.5
        signal_gene = true;
        else
        signal_gene = false;
        end
        %Mesure nombre de tours turbine
        if (~signal_gene_prec)&&(signal_gene)
        nb_tours=nb_tours + 1;
        end
        signal_gene_prec=signal_gene;
        %
        %Traitement évènement tension image de Upuiss
        if (image_Upuiss_prec<=0.2)&&(image_Upuiss > 0.2)
        send(when_image_Upuiss_sup_seuilHaut, Gestion_LEDS);
        elseif (image_Upuiss_prec>=0.18)&&(image_Upuiss< 0.18)
        send(when_image_Upuiss_inf_seuilBas, Gestion_LEDS);
        end
        image_Upuiss_prec=image_Upuiss;
        %Traitement évènement Ualim processeur<1.65V
        if (alim_LOW_prec==false)&&(alim_LOW==true)
        send(when_alim_low, Gestion_LEDS);
        end
        alim_LOW_prec=alim_LOW;
        %Gestion évènemts when_vol_eau_sup_xxl (seuils divisés par 10)
        if (nb_tours_prec<=5450)&&(nb_tours>5450)
        send(when_vol_eau_sup_10l, Gestion_LEDS);
        end
        if (nb_tours_prec<=10900)&&(nb_tours>10900)
        send(when_vol_eau_sup_20l, Gestion_LEDS);
        end
        if (nb_tours_prec<=16350)&&(nb_tours>16350)
        send(when_vol_eau_sup_30l, Gestion_LEDS);
        end
        if (nb_tours_prec<=21800)&&(nb_tours>21800)
        send(when_vol_eau_sup_40l, Gestion_LEDS);
        end
        nb_tours_prec=nb_tours;
        %
        %Gestion conditions vol_eau_sup_xxl
        vol_eau_sup_10l =(nb_tours>5450);
        vol_eau_sup_20l =(nb_tours>10900);
        vol_eau_sup_30l =(nb_tours>16350);
        vol_eau_sup_40l =(nb_tours>21800);
    state Gestion_LEDS [parallel]
      state Pommeau_OFF
        en : RGB=0b000;
        nb_tours=0;
        vol_eau_sup_10l=false; vol_eau_sup_20l=false;
        vol_eau_sup_30l=false; vol_eau_sup_40l=false;
      state eclairage_jets_d_eau
        state Vert
          RGB=0b010;
        state Bleu
          RGB=0b001;
        state Violet
          RGB=0b101;
        state Rouge
          RGB=0b100;
        state Rouge_clignotant
          state Rouge_1_seconde
            RGB=0b100;
          state Noir_1_seconde
            RGB=0b000;
          (default) -> Rouge_1_seconde
          Rouge_1_seconde -> Noir_1_seconde : after(1,sec)
          Noir_1_seconde -> Rouge_1_seconde : after(1,sec)
        (default) -> Vert
        Vert -> Bleu : when_vol_eau_sup_10l
        Bleu -> Violet : when_vol_eau_sup_20l
        Violet -> Rouge : when_vol_eau_sup_30l
        Rouge -> Rouge_clignotant : when_vol_eau_sup_40l
      state Pause
        RGB=0b000;
      (default) -> Pommeau_OFF
      Pommeau_OFF -> eclairage_jets_d_eau : when_image_Upuiss_sup_seuilHaut
      Pause -> Pommeau_OFF : when_alim_low
      eclairage_jets_d_eau -> Pause : when_image_Upuiss_inf_seuilBas
      (junction 294) -> eclairage_jets_d_eau
      (junction 294) -> Bleu : [vol_eau_sup_10l]
      (junction 293) -> (junction 294)
      (junction 293) -> Violet : [vol_eau_sup_20l]
      (junction 292) -> (junction 293)
      (junction 292) -> Rouge : [vol_eau_sup_30l]
      (junction 291) -> (junction 292)
      (junction 291) -> Rouge_clignotant : [vol_eau_sup_40l]
      Pause -> (junction 291) : when_image_Upuiss_sup_seuilHaut
  data: LED_R output; LED_V output; LED_B output; creneau_gene input =0; image_Upuiss input; signal_gene_prec local boolean; signal_gene local boolean; RGB local uint8; alim_LOW_prec local boolean; alim_LOW input boolean; image_Upuiss_prec local; nb_tours_prec local; vol_eau_sup_40l local; vol_eau_sup_10l local; vol_eau_sup_20l local; vol_eau_sup_30l local; nb_tours output
  events: local FUNCTION_CALL_EVENT; local FUNCTION_CALL_EVENT; local FUNCTION_CALL_EVENT; local FUNCTION_CALL_EVENT; local FUNCTION_CALL_EVENT; local FUNCTION_CALL_EVENT; local FUNCTION_CALL_EVENT
